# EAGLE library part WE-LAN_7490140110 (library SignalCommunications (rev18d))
WE-LAN LAN Transformer Characteristics Compliant with standards: IEEE 802.3u, IEEE 802.3ab, IEEE 802.3af, IEEE 802.3at and upcoming IEE 802.3bt SMD Applications Ethernet speed up to 10 Gbit/s Power over Ethernet PoE and PoE+ Compliant with most IC’s for Ethernet applications such as Intel, AMD, Microchip and Realtek Hub, Router, Switches, IPcameras, IoT Details see: http://katalog.we-online.de/en/pbs/WE-LAN/7490140110? Created by Yingchun Shan 2016 (C) Wurth Elektronik
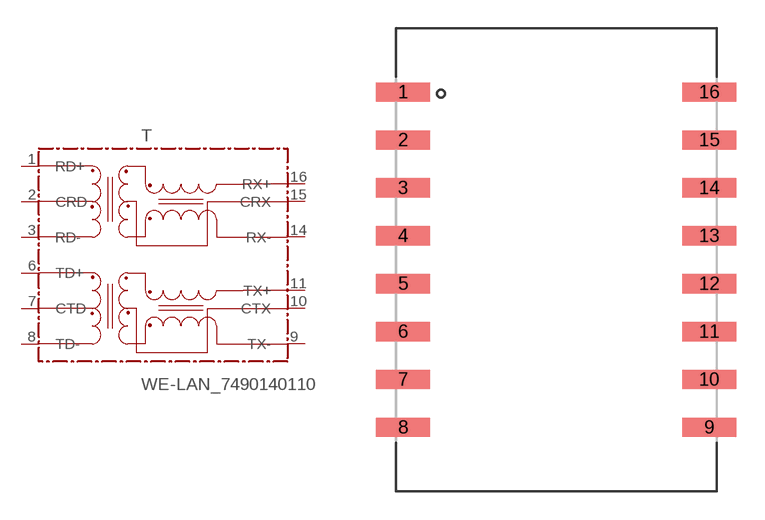
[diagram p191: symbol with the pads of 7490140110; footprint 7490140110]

Designator prefix T

## WE-LAN_7490140110  [7490140110]
1  RD+
2  CRD
3  RD-
6  TD+
7  CTD
8  TD-
9  TX-
10  CTX
11  TX+
14  RX-
15  CRX
16  RX+

## Footprint 7490140110 (pad centres in mm)
smd 2.87 x 1.02: 1 -8.115,8.89; 2 -8.115,6.35; 3 -8.115,3.81; 4 -8.115,1.27; 5 -8.115,-1.27; 6 -8.115,-3.81; 7 -8.115,-6.35; 8 -8.115,-8.89; 9 8.115,-8.89; 10 8.115,-6.35; 11 8.115,-3.81; 12 8.115,-1.27; 13 8.115,1.27; 14 8.115,3.81; 15 8.115,6.35; 16 8.115,8.89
